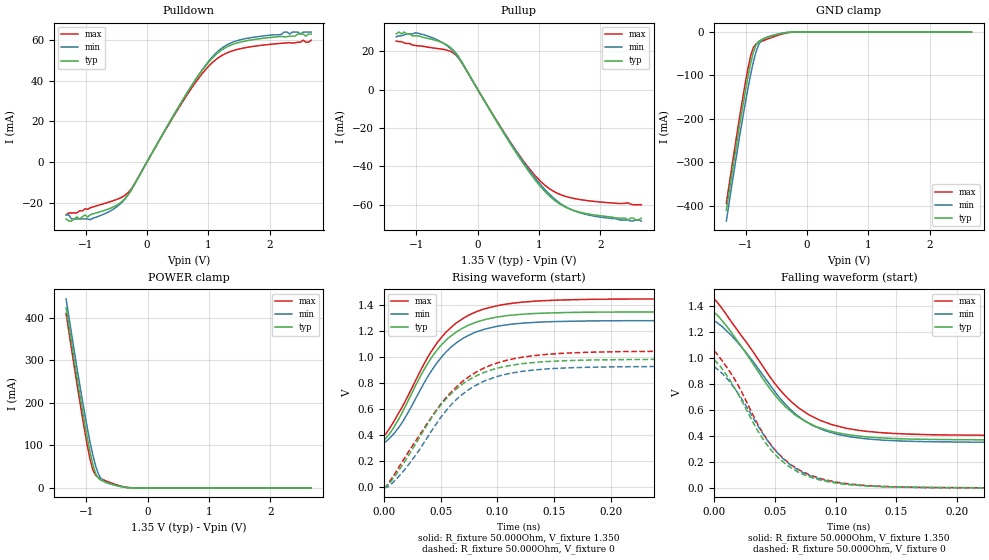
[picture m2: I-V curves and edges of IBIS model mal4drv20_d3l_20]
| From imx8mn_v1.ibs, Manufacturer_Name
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[Model] mal4drv20_d3l_20
Model_type   I/O
Polarity   Non-Inverting
Enable   Active-High
C_comp   1.688pF   1.681pF   1.696pF
C_comp_pullup   733.177fF   719.609fF   740.559fF
C_comp_pulldown 902.546fF   889.404fF   920.319fF
Vinh = 805.000mV
Vinl = 545.000mV
Vmeas = 675.000mV
Vref = 675.000mV
Rref = 50Ohms
Cref = 0pF
[Model Spec]
Vinh   805.000mV   772.000mV   855.000mV
Vinl   545.000mV   512.000mV   595.000mV
Vmeas   675.000mV   642.000mV   725.000mV
Vref   675.000mV   642.000mV   725.000mV
D_overshoot_ampl_h 0.4 NA   NA
D_overshoot_ampl_l 0.4 NA   NA
D_overshoot_area_l 110.000m NA   NA
D_overshoot_area_h 110.000m NA   NA
|[Receiver Thresholds]
|Vth = 675.000mV
|Vth_min = 642.000mV
|Vth_max = 725.000mV
|Vinh_ac = 150.000mV
|Vinh_dc = 100.000mV
|Vinl_ac = -150.000mV
|Vinl_dc = -100.000mV
|Tslew_ac = 5.000ns
|Threshold_sensitivity = 0.5
|Reference_supply Pullup_ref
[Temperature Range]   25.000   125.000   -40.000
[Voltage Range]   1.350V   1.283V   1.450V
[GND Clamp Reference]   0.00V   0.00V   0.00V
|[C Comp Corner]
|| variable   typ   min   max
|C_comp 1.696pF   1.681pF   1.688pF
|C_comp_pullup 740.559fF   719.609fF   733.177fF
|C_comp_pulldown 902.546fF   920.319fF   889.404fF
[Pulldown Reference]   0.00V   0.00V   0.00V
[POWER Clamp Reference]   1.350V   1.283V   1.450V
[Pullup Reference]   1.350V   1.283V   1.450V
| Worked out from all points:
|   slope of the pulldown table from 0 to 0.203 V, typ, clamps not added: 18.7 ohm
|   slope of the pullup table from 0 to 0.203 V, typ, clamps not added: 18.3 ohm
|   GND clamp passes 1 mA (typ) near -0.33 V on its own axis
|   POWER clamp passes 1 mA (typ) near -0.36 V on its own axis
|   rising waveform, R_fixture 50.000Ohm, V_fixture 1.350: 20-80 % time 42.1ps typ, 43.1ps min, 44.8ps max; typ from 0.361 V to 1.35 V
|   rising waveform, R_fixture 50.000Ohm, V_fixture 0: 20-80 % time 50.2ps typ, 50.8ps min, 56.1ps max; typ from -0.005 V to 0.985 V
|   falling waveform, R_fixture 50.000Ohm, V_fixture 1.350: 20-80 % time 48.8ps typ, 50ps min, 53.1ps max; typ from 1.35 V to 0.369 V
|   falling waveform, R_fixture 50.000Ohm, V_fixture 0: 20-80 % time 41.4ps typ, 43.1ps min, 42.5ps max; typ from 0.987 V to 0 V
[GND Clamp]
-1.318V   -410mA     -435mA     -394mA
-1.099V   -212mA     -238mA     -193mA
-1.011V   -139mA     -165mA     -119mA
-966.7mV  -104mA     -131mA     -84.77mA
-922.7mV  -73.08mA   -98.61mA   -55.67mA
-878.8mV  -47.18mA   -69.91mA   -36.06mA
-834.8mV  -29.86mA   -46.17mA   -27.79mA
-790.9mV  -21.59mA   -29.3mA    -24.32mA
-703mV    -15.41mA   -14.73mA   -19.21mA
-439.4mV  -3.973mA   -3.431mA   -5.961mA
-219.7mV  -62.42uA   -101.9uA   -153.4uA
2.68V     65.01nA    1.698uA    29.72nA
[Power Clamp]
-1.33V    424mA      444.5mA    410.3mA
-1.199V   302mA      324mA      287mA
-1.067V   186mA      208.6mA    168.5mA
-978.8mV  114mA      137.2mA    95.83mA
-934.8mV  81.28mA    104.7mA    64.68mA
-890.9mV  53.35mA    75.52mA    41.63mA
-847mV    33.16mA    50.86mA    29.5mA
-803mV    22.54mA    32.62mA    24.29mA
-715.2mV  15.14mA    15.5mA     18.5mA
-495.5mV  4.953mA    4.871mA    6.554mA
-275.8mV  132.3uA    356.2uA    190.3uA
2.668V    -205nA     -2.419uA   -83.46nA
[Pulldown]
-1.318V   -28mA      -26mA      -26mA
-1.23V    -29mA      -28mA      -25mA
-922.7mV  -25.88mA   -28.39mA   -22.46mA
-571.2mV  -22.4mA    -23.62mA   -19.22mA
-395.5mV  -19.12mA   -19.46mA   -17.06mA
-219.7mV  -11.93mA   -11.89mA   -11.59mA
747mV     38.34mA    38.49mA    37.2mA
966.7mV   47.68mA    48.09mA    45.85mA
1.186V    54.42mA    55.25mA    51.77mA
1.626V    59.71mA    60.86mA    56.42mA
2.241V    61.65mA    64mA       58.57mA
2.68V     63mA       64mA       60mA
[Pullup]
-1.33V    29mA       27.53mA    25.28mA
-1.199V   30mA       28.52mA    24.28mA
-978.8mV  28mA       29.48mA    22.81mA
-627.3mV  25.07mA    25.39mA    21.28mA
-407.6mV  20.88mA    20.2mA     19.24mA
-275.8mV  15.32mA    14.81mA    14.74mA
734.8mV   -38.23mA   -37.32mA   -36.75mA
998.5mV   -49.61mA   -48.55mA   -47.01mA
1.262V    -58mA      -57.27mA   -53.49mA
1.746V    -64.51mA   -64.94mA   -57.72mA
2.449V    -68mA      -68mA      -59.06mA
2.668V    -67mA      -68.53mA   -60mA
[Ramp]
R_load=50.000Ohm
dV/dt_r   589.800mV/47.000ps  558.899mV/48.000ps  628.200mV/51.500ps
dV/dt_f   589.800mV/46.500ps  558.899mV/47.500ps  628.200mV/48.500ps
[Rising waveform]
R_fixture=50.000Ohm
V_fixture=1.350
V_fixture_min=1.283
V_fixture_max=1.450
0s        361mV      347mV      403mV
4ps       401mV      368mV      439mV
14ps      539mV      471mV      585mV
37ps      930mV      826mV      974mV
50ps      1.089V     993mV      1.145V
70ps      1.226V     1.147V     1.301V
92ps      1.296V     1.223V     1.381V
122ps     1.331V     1.263V     1.425V
166ps     1.346V     1.278V     1.444V
469ps     1.35V      1.283V     1.45V
[Rising waveform]
R_fixture=50.000Ohm
V_fixture=0
0s        -5.408mV   -33.58uV   -4.281mV
4ps       21.91mV    6.153mV    29.67mV
17ps      179mV      121mV      209mV
44ps      560mV      460mV      566mV
58ps      709mV      622mV      720mV
79ps      847mV      775mV      873mV
107ps     929mV      868mV      974mV
140ps     965mV      908mV      1.02V
185ps     979mV      924mV      1.04V
470ps     985mV      930mV      1.048V
[Falling waveform]
R_fixture=50.000Ohm
V_fixture=1.350
V_fixture_min=1.283
V_fixture_max=1.450
0s        1.352V     1.287V     1.456V
18ps      1.148V     1.136V     1.229V
47ps      751mV      779mV      842mV
59ps      623mV      641mV      706mV
70ps      542mV      547mV      613mV
81ps      485mV      481mV      549mV
107ps     414mV      403mV      463mV
136ps     386mV      370mV      426mV
179ps     373mV      355mV      409mV
469ps     369mV      351mV      404mV
[Falling waveform]
R_fixture=50.000Ohm
V_fixture=0
0s        987mV      933mV      1.055V
7ps       913mV      879mV      975mV
16ps      785mV      779mV      852mV
36ps      439mV      479mV      490mV
48ps      280mV      315mV      316mV
65ps      145mV      162mV      168mV
88ps      58.88mV    65.37mV    70.12mV
110ps     25.23mV    27.87mV    30.95mV
155ps     4.737mV    5.601mV    6.187mV
469ps     10.17uV    14.54uV    11.37uV
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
